// 事件处理对象的实例
VAR_GLOBAL
	FB_EventloggerHandlingProductionInfo  : FB_EventloggerHandlingExtend(TC_Events.MyEvent.ProductionInfo1) ;
	FB_EventloggerHandlingAxisPosition    : FB_EventloggerHandlingExtend(TC_Events.MyEvent.AxisPosition) ;
	FB_EventloggerHandlingCylinderTemp    : FB_EventloggerHandlingExtend(TC_Events.MyEvent.CylinderTemp) ;
	
	//FB_EventloggerHandlingMyEvent   	  : FB_EventloggerHandlingExtend(TC_Events.MyEvent.) ;
END_VAR
